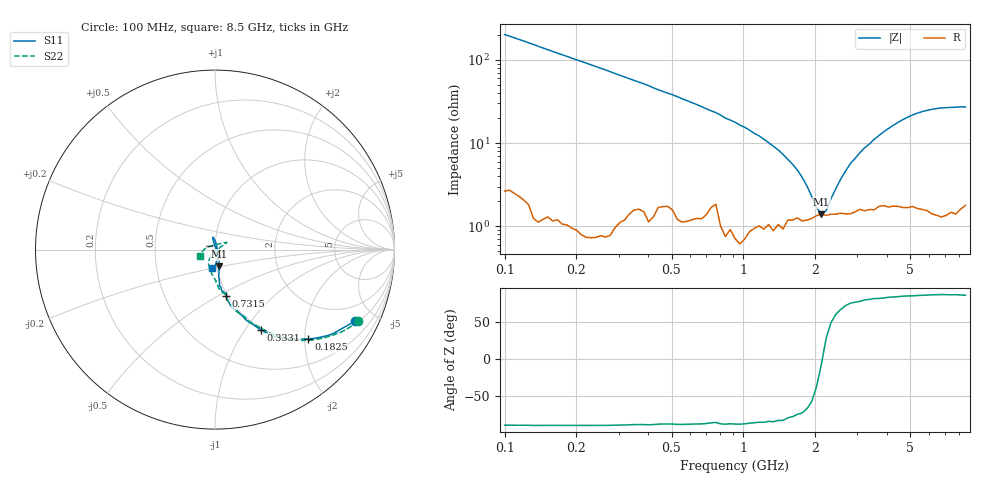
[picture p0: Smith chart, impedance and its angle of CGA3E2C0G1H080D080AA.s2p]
! S-parameter Generated by TDK Corporation
! Copyright(C) 2015 TDK Corporation.
! All Rights Reserved.
! TDK P/N: CGA3E2C0G1H080D080AA (Multilayer Ceramic Chip Capacitors)
! Property: C=8pF
! Size(LxWxT): 1.6x0.8x0.8mm, 0.063x0.031x0.031inches
! Model Type: s2p (Touchstone File Format Version 1.0)
! Frequency: DC=Yes Start=100MHz Stop=8500MHz 98points Log-sweep
! Note:
! Model Generated on Jun. 23, 2015
! Hash(MD5):
! Port Assignments:
!  1 ---| |--- 2
! Applicable Conditions:
!  Temperature = 25 degC
!  DC Bias Voltage = 0 V
!  Small Signal Operation
! Terms and conditions regarding TDK Simulation Models
! (1)This simulation model is being provided solely for informational purposes. Please refer to the specifications of the products in terms of detailed characteristics of such products.
! (2)In no event shall TDK Corporation of any of its subsidiaries be liable for any loss or damage arising, directly or indirectly,
!  From any information contained in this simulation model, including, but not limited to loss or damages arising from any inaccuracies, omissions or errors in connection with such information.
! (3)Any and all copyrights on this simulation model are owned by TDK Corporation.
!  Duplication or redistribution of this simulation model without prior written permission from TDK Corporation is prohibited.
! (4)This simulation model is subject to any modification or change without any prior notice.
! (5)Neither TDK Corporation nor any of its subsidiaries shall make any warranty, express or implied,
!  Including but not limited to the correctness, implied warranties of merchantability and fitness for a particular purpose with respect to this simulation models.
! (6)The use of this simulation model shall be deemed to have consented to the terms and conditions hereof.
# MHz S MA R 50
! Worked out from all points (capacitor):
!   97 points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, 100 MHz to 8.5 GHz, reference 50 ohm
!   read as one part in series: C = 7.82 pF near 100 MHz
!   lowest |Z| = 1.4 ohm at 2.121 GHz (marker M1)
!   series resonance near 2.139 GHz, so ESL is about 710 pH
!   S11 on the Smith chart (normalised r, x): 100 MHz: 1.13, -3.83; 182.5 MHz: 1.01, -2.08; 333.1 MHz: 0.98, -1.19; 731.5 MHz: 0.98, -0.55; 8.5 GHz: 0.95, -0.20
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100  0.874 -27.1  0.4343 62.6  0.4338 62.6  0.8929 -26.5
182.5053  0.7198 -43.7  0.6554 46.8  0.6557 46.7  0.7429 -42.6
333.0818  0.516 -60.1  0.8394 29.3  0.8389 29.4  0.5102 -59.5
482.3207  0.372 -69.5  0.8996 20.0  0.8999 20.0  0.3891 -68.1
731.5077  0.2661 -76.4  0.9406 11.5  0.9419 11.5  0.2602 -76.8
1533.871  0.1345 -80.9  0.9701 -0.6  0.9707 -0.5  0.1298 -98.3
2120.682  0.09675 -75.4  0.9716 -5.2  0.9719 -5.2  0.09557 -110.4
2931.989  0.05337 -69.6  0.9725 -10.3  0.9727 -10.2  0.05661 -120.1
3368.656  0.02745 -61.5  0.9734 -12.7  0.9729 -12.7  0.03185 -115.7
3695.327  0.007122 -36.9  0.9715 -14.5  0.9714 -14.5  0.01181 -72.7
3870.357  0.01255 63.1  0.9706 -15.5  0.9714 -15.4  0.01146 -21.4
4053.677  0.01946 96.1  0.9714 -16.5  0.9704 -16.4  0.02242 14.1
4245.68  0.03207 94.9  0.9697 -17.4  0.9696 -17.4  0.03255 25.1
4446.777  0.04152 100.5  0.9697 -18.6  0.9697 -18.5  0.04655 27.0
5109.044  0.06691 100.2  0.967 -22.0  0.9643 -21.9  0.07518 31.5
5869.945  0.06491 96.8  0.9644 -25.7  0.9646 -25.7  0.07046 33.3
6439.175  0.0425 84.9  0.9651 -28.5  0.9643 -28.4  0.04613 47.5
6744.168  0.02198 65.7  0.9646 -30.0  0.9685 -30.1  0.03164 67.8
7063.606  0.01535 -11.8  0.9649 -31.6  0.9628 -31.5  0.02599 113.4
7398.175  0.03566 -62.4  0.963 -33.2  0.9613 -33.3  0.03658 152.9
7748.59  0.06084 -79.5  0.9595 -35.2  0.961 -35.0  0.05692 175.4
8500  0.1066 -99.0  0.9555 -39.3  0.9553 -38.9  0.09123 -155.9
